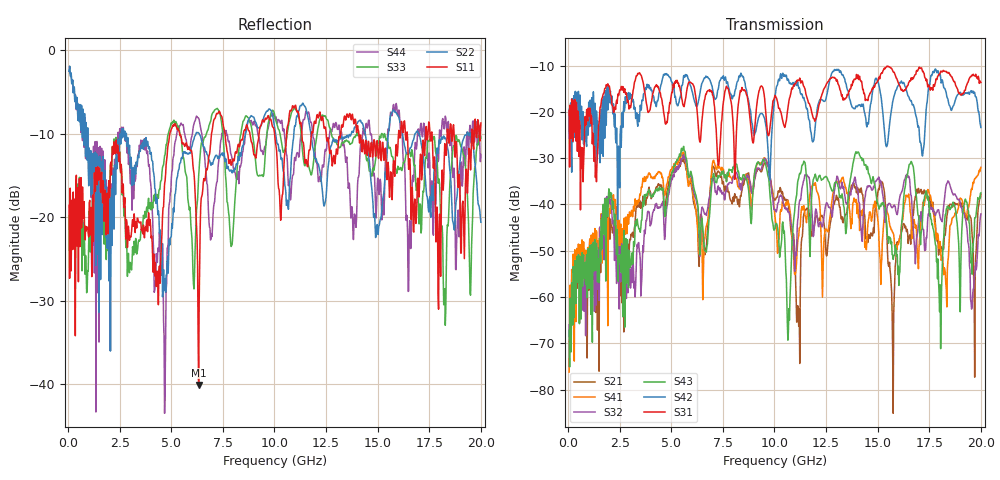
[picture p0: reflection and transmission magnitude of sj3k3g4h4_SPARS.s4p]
! FILE: E:\users\goganessyan\GBX_Backplane\FR408_backplane\1m_INBOUND_NEXT\sj3k3g4h4_SPARS.s4p
# MHZ S RI R 50.00
! FREQ  S11  S12  S13  S14
!  S21  S22  S23  S24
!  S31  S32  S33  S34
!  S41  S42  S43  S44
!  REAL  IMAG  REAL  IMAG  REAL  IMAG  REAL  IMAG
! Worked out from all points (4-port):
!   799 points, 50 MHz to 20 GHz, reference 50 ohm
!   strongest paths, dB at 50 MHz, 5.025 GHz, 10.03 GHz, 15.03 GHz, 20 GHz:
!     S31: -19.7, -15.8, -16.5, -13.2, -13.7
!     S42: -19.4, -13.6, -16.7, -13.6, -23.4
!     S43: -67.2, -33.5, -45.2, -40.3, -37.5
!     S32: -66.0, -34.2, -41.1, -34.5, -42.0
!     S41: -76.2, -32.5, -42.6, -44.0, -32.0
!     S21: -69.6, -33.1, -39.1, -36.9, -37.8
!   lowest |S11| = -40.1 dB at 6.325 GHz (marker M1), VSWR 1.02, Z = 49.1 - j0.283 ohm
!   |S11| at or under -10 dB: start of sweep to 4.93 GHz; 5.404 GHz to 6.948 GHz (1.543 GHz wide, 25 % of centre); 14.09 GHz to 16.01 GHz (1.926 GHz wide, 12.8 % of centre)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
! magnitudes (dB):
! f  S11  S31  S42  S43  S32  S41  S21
! 50 MHz  -18.6  -19.7  -19.4  -67.2  -66.0  -76.2  -69.6
! 4.7 GHz  -15.6  -22.4  -11.7  -42.6  -46.7  -37.8  -41.5
! 6.325 GHz  -40.1  -24.5  -17.5  -43.1  -43.2  -50.7  -51.2
! 11.15 GHz  -7.3  -13.2  -14.4  -34.6  -42.8  -47.2  -63.4
! 15.2 GHz  -12.2  -11.6  -18.1  -39.8  -36.3  -51.6  -35.1
! 15.75 GHz  -13.7  -11.4  -17.3  -51.9  -40.5  -46.2  -85.1
! 20 GHz  -8.7  -13.7  -23.4  -37.5  -42.0  -32.0  -37.8
